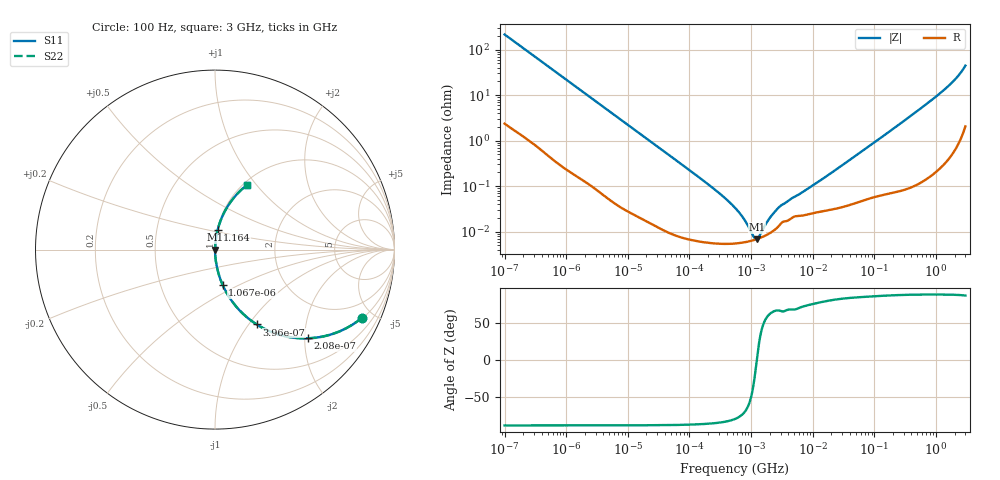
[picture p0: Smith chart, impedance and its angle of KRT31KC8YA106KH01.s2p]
!Murata Part Number: KRT31KC8YA106KH01
!These Parameters are Measured in Series Mode Connection
!Data Generated on Jan 08, 2026
!  o--ll--o
!Port1  Port2
!  o------o
!Operation Temp=25[degC], DC Bias Voltage=0[V]
!Freq. Start=100[Hz] Stop=3[GHz] 401[Steps]
# Hz S RI R 50
!Freq.(Hz) S11(Real) S11(Imag) S21(Real) S21(Imag) S12(Real) S12(Imag) S22(Real) S22(Imag)
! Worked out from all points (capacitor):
!   401 points, 100 Hz to 3 GHz, reference 50 ohm
!   read as one part in series: C = 7.4 uF near 109 Hz
!   lowest |Z| = 6.84 mohm at 1.241 MHz (marker M1)
!   series resonance near 1.236 MHz, so ESL is about 2.2 nH
!   S11 on the Smith chart (normalised r, x): 100 Hz: 1.05, -4.30; 208 Hz: 1.02, -2.08; 396 Hz: 1.01, -1.10; 1.067 kHz: 1.00, -0.41; 1.164 GHz: 1.00, +0.22; 3 GHz: 1.04, +0.89
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100  0.8192 -0.3794  0.1808 0.3794  0.1808 0.3794  0.8192 -0.3794
208  0.5188 -0.494  0.4812 0.494  0.4812 0.494  0.5188 -0.494
396  0.2332 -0.4173  0.7668 0.4173  0.7668 0.4173  0.2332 -0.4173
636  0.1073 -0.3043  0.8927 0.3043  0.8927 0.3043  0.1073 -0.3043
1067  0.0421 -0.1956  0.9579 0.1956  0.9579 0.1956  0.0421 -0.1956
1788  0.0161 -0.1204  0.9839 0.1204  0.9839 0.1204  0.0161 -0.1204
5476  0.00208 -0.0402  0.9979 0.0402  0.9979 0.0402  0.00208 -0.0402
31977  0.000169 -0.00699  0.9998 0.00699  0.9998 0.00699  0.000169 -0.00699
231582  5.64e-05 -0.000941  0.9999 0.000941  0.9999 0.000941  5.64e-05 -0.000941
547723  5.48e-05 -0.00033  0.9999 0.00033  0.9999 0.00033  5.48e-05 -0.00033
709116  5.7e-05 -0.000212  0.9999 0.000212  0.9999 0.000212  5.7e-05 -0.000212
1000599  6.27e-05 -7.67e-05  0.9999 7.67e-05  0.9999 7.67e-05  6.27e-05 -7.67e-05
1240863  6.84e-05 1.3e-06  0.9999 -1.3e-06  0.9999 -1.3e-06  6.84e-05 1.3e-06
1411895  7.31e-05 4.74e-05  0.9999 -4.74e-05  0.9999 -4.74e-05  7.31e-05 4.74e-05
1538820  7.67e-05 7.82e-05  0.9999 -7.82e-05  0.9999 -7.82e-05  7.67e-05 7.82e-05
2079876  9.51e-05 0.00019  0.9999 -0.00019  0.9999 -0.00019  9.51e-05 0.00019
2934810  0.000142 0.00033  0.9999 -0.00033  0.9999 -0.00033  0.000142 0.00033
9794414  0.000252 0.000983  0.9997 -0.000983  0.9997 -0.000983  0.000252 0.000983
1.751444e8  0.000932 0.0157  0.9991 -0.0157  0.9991 -0.0157  0.000932 0.0157
1.163803e9  0.0142 0.1078  0.9858 -0.1078  0.9858 -0.1078  0.0142 0.1078
2.126076e9  0.0582 0.22  0.9418 -0.22  0.9418 -0.22  0.0582 0.22
3e9  0.1758 0.3582  0.8242 -0.3582  0.8242 -0.3582  0.1758 0.3582
